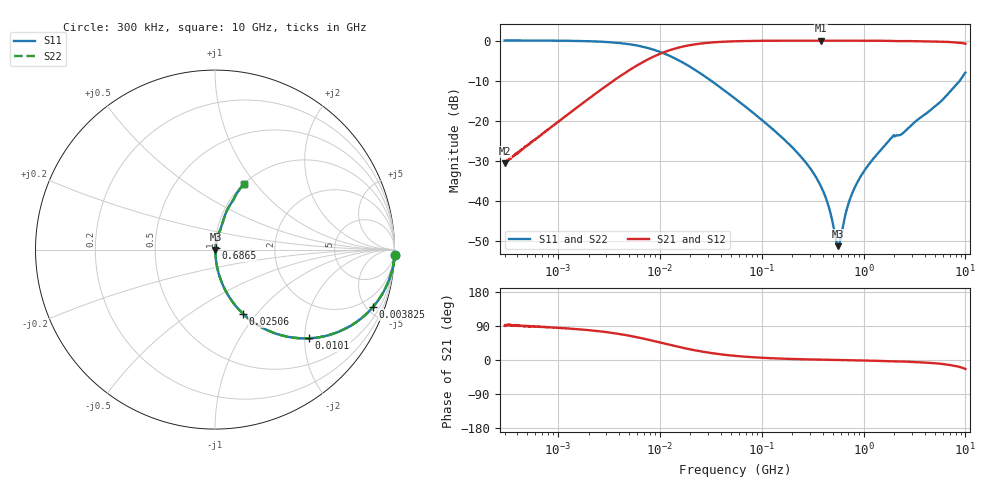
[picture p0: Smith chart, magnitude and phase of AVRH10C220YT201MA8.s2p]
! S-Parameter Data Generated by TDK Corporation
! Copyright(C) 2023 TDK Corporation.
! All Rights Reserved.
! TDK P/N: AVRH10C220YT201MA8 (Varistor)
! Property: V1mA=22V
! Size(LxWxT): 1x0.5x0.5mm
! Model Type: s2p (Touchstone File Format Version 1.0)
! Frequency: DC=Yes Start=0.3MHz Stop=10000MHz 1602points Log-sweep
! Model Generated on Oct. 12, 2023
! Port Assignments:
!  1 ---N--- 2
! Applicable Conditions:
!  Temperature = 25 degC
!  DC Bias Voltage = 0 V
!  Small Signal Operation
! Terms and conditions regarding TDK Simulation Models
! (1)This simulation model is being provided solely for informational purposes. Please refer to the specifications of the products in terms of detailed characteristics of such products.
! (2)In no event shall TDK Corporation of any of its subsidiaries be liable for any loss or damage arising, directly or indirectly,
!  From any information contained in this simulation model, including, but not limited to loss or damages arising from any inaccuracies, omissions or errors in connection with such information.
! (3)Any and all copyrights on this simulation model are owned by TDK Corporation.
!  Duplication or redistribution of this simulation model without prior written permission from TDK Corporation is prohibited.
! (4)This simulation model is subject to any modification or change without any prior notice.
! (5)Neither TDK Corporation nor any of its subsidiaries shall make any warranty, express or implied,
!  Including but not limited to the correctness, implied warranties of merchantability and fitness for a particular purpose with respect to this simulation models.
! (6)The use of this simulation model shall be deemed to have consented to the terms and conditions hereof.
# Hz S MA R 50
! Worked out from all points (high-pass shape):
!   1601 points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, 300 kHz to 10 GHz, reference 50 ohm
!   highest |S21| = -0.02 dB at 381.7 MHz (marker M1); lowest = -30.6 dB at 302.3 kHz (marker M2)
!   |S21| within 3 dB of the highest: 10.71 MHz to end of sweep
!   lowest |S11| = -51.2 dB at 562.7 MHz (marker M3), VSWR 1.01, Z = 50.3 - j0.0114 ohm
!   |S11| at or under -10 dB: 31.85 MHz to 8.815 GHz (8.783 GHz wide, 199 % of centre)
!   |S22| runs from -51.2 to 0.0 dB; largest |S21 - S12| = 0
!   S11 on the Smith chart (normalised r, x): 300 kHz: -1, -66; 3.825 MHz: 1.06, -5.50; 10.1 MHz: 1.02, -2.10; 25.06 MHz: 1.01, -0.85; 686.5 MHz: 1.01, +0.01; 10 GHz: 1.01, +0.87
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300000  1.001 -1.7  0.03021 90.3  0.03021 90.3  1.001 -1.7
302300  1.001 -1.7  0.0294 91.8  0.0294 91.8  1.001 -1.7
1702534  0.9861 -9.3  0.161 80.4  0.161 80.4  0.9861 -9.3
3825302  0.9364 -19.9  0.3403 69.4  0.3403 69.4  0.9364 -19.9
9678464  0.7352 -42.1  0.6699 47.3  0.6699 47.3  0.7352 -42.1
1.009555e7  0.7209 -43.2  0.6852 46.1  0.6852 46.1  0.7209 -43.2
2.506097e7  0.3898 -66.4  0.9166 22.9  0.9166 22.9  0.3898 -66.4
5.477226e7  0.1897 -78.2  0.9791 10.9  0.9791 10.9  0.1897 -78.2
1.676739e8  0.05802 -84.5  0.9962 3.3  0.9962 3.3  0.05802 -84.5
3.128687e8  0.02366 -83.1  0.9974 1.3  0.9974 1.3  0.02366 -83.1
3.817091e8  0.01529 -80.0  0.9975 0.9  0.9975 0.9  0.01529 -80.0
4.51086e8  0.008878 -72.6  0.9974 0.5  0.9974 0.5  0.008878 -72.6
5.344909e8  0.003387 -37.2  0.9973 0.1  0.9973 0.1  0.003387 -37.2
5.627284e8  0.002743 -2.4  0.9973 0.0  0.9973 0.0  0.002743 -2.4
5.916e8  0.0033 32.2  0.9972 -0.1  0.9972 -0.1  0.0033 32.2
6.86464e8  0.00797 67.8  0.997 -0.4  0.997 -0.4  0.00797 67.8
7.449157e8  0.011 73.2  0.9969 -0.6  0.9969 -0.6  0.011 73.2
9.505123e8  0.02086 79.1  0.9963 -1.2  0.9963 -1.2  0.02086 79.1
1.767627e9  0.05629 79.0  0.9908 -3.2  0.9908 -3.2  0.05629 79.0
2.417222e9  0.06958 75.5  0.9849 -3.9  0.9849 -3.9  0.06958 75.5
5.531592e9  0.1672 74.0  0.9673 -9.6  0.9673 -9.6  0.1672 74.0
1e10  0.3997 66.0  0.9135 -23.6  0.9135 -23.6  0.3997 66.0
